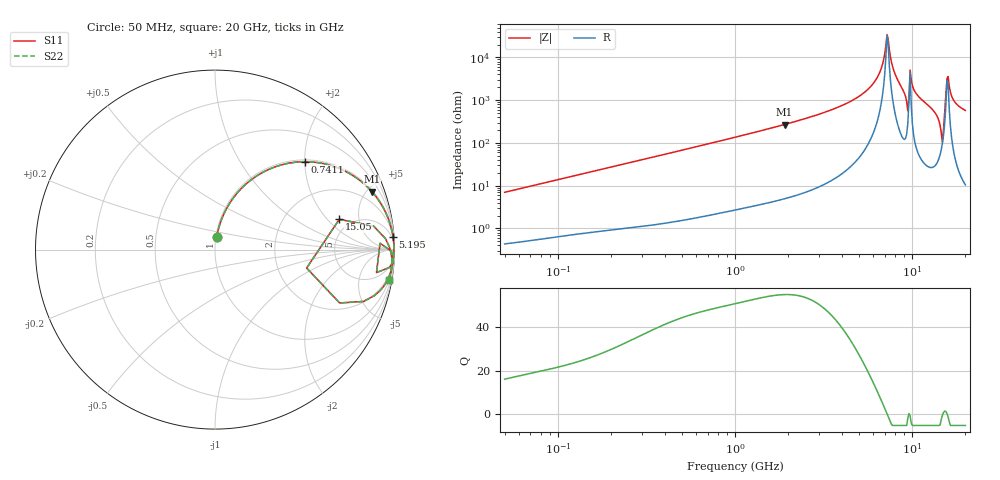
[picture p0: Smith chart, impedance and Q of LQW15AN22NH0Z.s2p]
!Murata Part Number: LQW15AN22NH0Z
!These Parameters are Measured in Series Mode Connection
!  o--[Z]--o
!Port1  Port2
!  o-------o
!Freq. Start=50[MHz] Stop=20[GHz], 401[Steps]
# Hz S RI R 50
!Freq.(Hz) S11(Real) S11(Imag) S21(Real) S21(Imag) S12(Real) S12(Imag) S22(Real) S22(Imag)
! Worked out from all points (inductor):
!   401 points, 50 MHz to 20 GHz, reference 50 ohm
!   read as one part in series: L = 22.1 nH near 51.52 MHz
!   highest Q = 54.7 at 1.904 GHz (marker M1), where L = 22.5 nH
!   self-resonance near 7.222 GHz
!   S11 on the Smith chart (normalised r, x): 50 MHz: 1.01, +0.14; 741.1 MHz: 1.04, +2.00; 5.195 GHz: 2, +27; 15.05 GHz: 4.00, +2.74; 20 GHz: 1, -11
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5e7  0.00908 0.0688  0.9909 -0.0688  0.9909 -0.0688  0.00908 0.0688
1.364002e8  0.0403 0.1773  0.9597 -0.1773  0.9597 -0.1773  0.0403 0.1773
3.721004e8  0.2069 0.3927  0.7931 -0.3927  0.7931 -0.3927  0.2069 0.3927
7.411344e8  0.4997 0.4897  0.5003 -0.4897  0.5003 -0.4897  0.4997 0.4897
1e9  0.6448 0.4688  0.3552 -0.4688  0.3552 -0.4688  0.6448 0.4688
1.904239e9  0.8746 0.3221  0.1254 -0.3221  0.1254 -0.3221  0.8746 0.3221
2.728004e9  0.9416 0.2251  0.0584 -0.2251  0.0584 -0.2251  0.9416 0.2251
5.194772e9  0.9917 0.0727  0.00825 -0.0727  0.00825 -0.0727  0.9917 0.0727
6.311513e9  0.9963 0.0306  0.00371 -0.0306  0.00371 -0.0306  0.9963 0.0306
6.701223e9  0.9969 0.0176  0.00306 -0.0176  0.00306 -0.0176  0.9969 0.0176
7.114996e9  0.9972 0.00426  0.00277 -0.00426  0.00277 -0.00426  0.9972 0.00426
7.442007e9  0.9972 -0.00602  0.00281 0.00602  0.00281 0.00602  0.9972 -0.00602
7.901521e9  0.9967 -0.0205  0.00329 0.0205  0.00329 0.0205  0.9967 -0.0205
9.316812e9  0.9722 -0.0996  0.0278 0.0996  0.0278 0.0996  0.9722 -0.0996
1.004137e10  0.9922 -0.0447  0.00776 0.0447  0.00776 0.0447  0.9922 -0.0447
1.066139e10  0.9909 -0.0733  0.00912 0.0733  0.00912 0.0733  0.9909 -0.0733
1.417136e10  0.8885 -0.2562  0.1115 0.2562  0.1115 0.2562  0.8885 -0.2562
1.460232e10  0.6943 -0.2973  0.3057 0.2973  0.3057 0.2973  0.6943 -0.2973
1.504638e10  0.6927 0.1686  0.3073 -0.1686  0.3073 -0.1686  0.6927 0.1686
1.597544e10  0.9813 -0.0202  0.0187 0.0202  0.0187 0.0202  0.9813 -0.0202
1.747767e10  0.9824 -0.1093  0.0176 0.1093  0.0176 0.1093  0.9824 -0.1093
2e10  0.9677 -0.1679  0.0323 0.1679  0.0323 0.1679  0.9677 -0.1679
